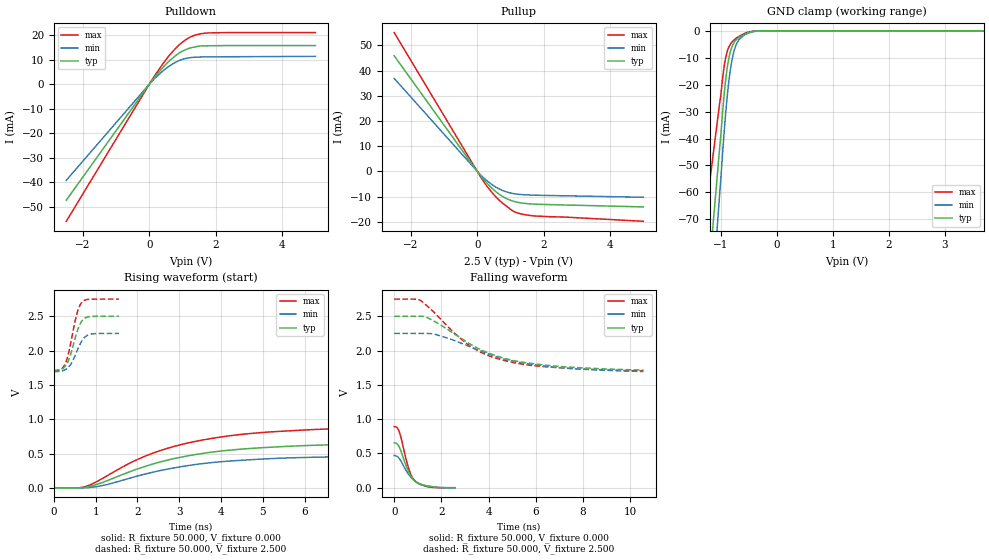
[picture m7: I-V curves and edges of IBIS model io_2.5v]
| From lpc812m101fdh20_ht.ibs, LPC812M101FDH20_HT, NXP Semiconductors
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[Model]   io_2.5v
Model_type I/O
Vinl=7.500E-01
Vinh=1.750E+00
Vref=0.000E+00
Rref=1.000E+06
Cref=2.000E-11
Vmeas=1.250E+00
C_comp   6.740E-13   6.620E-13   6.860E-13
[Voltage Range]   2.500E+00   2.250E+00   2.750E+00
[POWER Clamp Reference]   2.500E+00   2.250E+00   2.750E+00
[GND Clamp Reference]   0.000E+00   0.000E+00   0.000E+00
[Pullup Reference]   2.500E+00   2.250E+00   2.750E+00
[Pulldown Reference]   0.000E+00   0.000E+00   0.000E+00
[Temperature Range]   25   105   -40
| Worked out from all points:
|   slope of the pulldown table from 0 to 0.375 V, typ, clamps not added: 59.6 ohm
|   slope of the pullup table from 0 to 0.375 V, typ, clamps not added: 64.1 ohm
|   GND clamp passes 1 mA (typ) near -0.55 V on its own axis
|   rising waveform, R_fixture 50.000, V_fixture 0.000: 20-80 % time 2.43ns typ, 2.43ns min, 2.42ns max; typ from 0 V to 0.654 V
|   falling waveform, R_fixture 50.000, V_fixture 0.000: 20-80 % time 492ps typ, 580ps min, 423ps max; typ from 0.654 V to 0 V
|   rising waveform, R_fixture 50.000, V_fixture 2.500: 20-80 % time 235ps typ, 261ps min, 222ps max; typ from 1.72 V to 2.5 V
|   falling waveform, R_fixture 50.000, V_fixture 2.500: 20-80 % time 2.72ns typ, 3.09ns min, 2.36ns max; typ from 2.5 V to 1.72 V
[GND Clamp]
-2.5V     -400.8mA   -480.7mA   -270.8mA
-1.02V    -43.1mA    -60.31mA   -26.6mA
-1V       -38.68mA   -54.9mA    -23.79mA
-960mV    -28.15mA   -42.98mA   -16.18mA
-920mV    -19.39mA   -32.21mA   -10.63mA
-880mV    -12.91mA   -23.14mA   -7.24mA
-820mV    -7.048mA   -13.16mA   -4.672mA
-780mV    -4.938mA   -8.808mA   -3.728mA
-720mV    -3.192mA   -4.874mA   -2.627mA
-580mV    -1.272mA   -1.617mA   -998.7uA
-300mV    0A         0A         0A
5V        0A         0A         0A
[POWER Clamp]
-2.5V     0A         0A         0A
5V        0A         0A         0A
[Pullup]
-2.5V     45.89mA    36.9mA     55.11mA
140mV     -2.352mA   -1.91mA    -2.969mA
360mV     -5.652mA   -4.429mA   -7.051mA
580mV     -8.283mA   -6.419mA   -10.43mA
820mV     -10.42mA   -7.9mA     -13.24mA
1.04V     -11.68mA   -8.725mA   -15.48mA
1.32V     -12.55mA   -9.213mA   -16.91mA
1.72V     -13.01mA   -9.465mA   -17.72mA
5V        -14.13mA   -10.3mA    -19.84mA
[Pulldown]
-2.5V     -47.41mA   -39.28mA   -56.02mA
120mV     2.161mA    1.747mA    2.601mA
580mV     9.226mA    7.226mA    11.39mA
840mV     12.16mA    9.303mA    15.31mA
1.06V     13.92mA    10.4mA     17.85mA
1.38V     15.21mA    11.01mA    20.05mA
1.76V     15.68mA    11.14mA    20.93mA
5V        15.77mA    11.36mA    21.08mA
[Rising Waveform]
R_fixture = 50.000
V_fixture = 0.000
V_fixture_min = 0.000
V_fixture_max = 0.000
|  time   V(typ)   V(min)   V(max)
0s        0V         0V         0V
760ps     10.29mV    1.264mV    19.21mV
1.26ns    100.5mV    46.77mV    170.3mV
1.84ns    239.9mV    144.2mV    366.9mV
2.38ns    349.4mV    229.8mV    507.9mV
3.1ns     454.3mV    313.8mV    638.8mV
4.04ns    539.5mV    382.6mV    744.9mV
4.96ns    584mV      418.9mV    805.5mV
6.44ns    624mV      448.8mV    855.3mV
9.9ns     654.1mV    474.3mV    890.6mV
[Falling Waveform]
R_fixture = 50.000
V_fixture = 0.000
V_fixture_min = 0.000
V_fixture_max = 0.000
|  time   V(typ)   V(min)   V(max)
0s        654.1mV    469.6mV    890.6mV
120ps     640.5mV    456.8mV    876.6mV
200ps     603.7mV    431.9mV    829.6mV
280ps     541.1mV    391.8mV    741mV
600ps     243.2mV    200.4mV    294.8mV
720ps     165.8mV    148.4mV    180.9mV
860ps     103.5mV    100mV      106.7mV
1.1ns     53.65mV    48.2mV     51.15mV
1.46ns    21.75mV    20.79mV    11.23mV
2.58ns    0V         -2.224mV   0V
[Rising Waveform]
R_fixture = 50.000
V_fixture = 2.500
V_fixture_min = 2.250
V_fixture_max = 2.750
|  time   V(typ)   V(min)   V(max)
0s        1.717V     1.694V     1.706V
180ps     1.73V      1.702V     1.731V
280ps     1.779V     1.725V     1.818V
380ps     1.903V     1.779V     2.035V
560ps     2.282V     2.002V     2.554V
620ps     2.377V     2.083V     2.654V
680ps     2.439V     2.149V     2.709V
780ps     2.484V     2.214V     2.742V
900ps     2.498V     2.241V     2.749V
1.56ns    2.5V       2.25V      2.75V
[Falling Waveform]
R_fixture = 50.000
V_fixture = 2.500
V_fixture_min = 2.250
V_fixture_max = 2.750
|  time   V(typ)   V(min)   V(max)
0s        2.5V       2.25V      2.75V
1.1ns     2.5V       2.25V      2.733V
1.34ns    2.49V      2.25V      2.667V
1.7ns     2.426V     2.24V      2.554V
3.02ns    2.138V     2.082V     2.115V
3.64ns    2.017V     1.997V     1.98V
4.4ns     1.915V     1.902V     1.881V
5.46ns    1.829V     1.818V     1.8V
6.66ns    1.779V     1.762V     1.757V
10.56ns   1.717V     1.694V     1.706V
[Ramp]
dV/dt_r   3.9102E-01/2.4259E-09   2.8308E-01/2.4231E-09   5.3455E-01/2.4220E-09
dV/dt_f   4.7003E-01/2.7127E-09   3.3371E-01/3.0825E-09   6.2651E-01/2.3493E-09
R_load = 50
